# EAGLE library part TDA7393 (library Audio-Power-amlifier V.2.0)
2 x 35W Dual Bridge Car Radio Amplifier
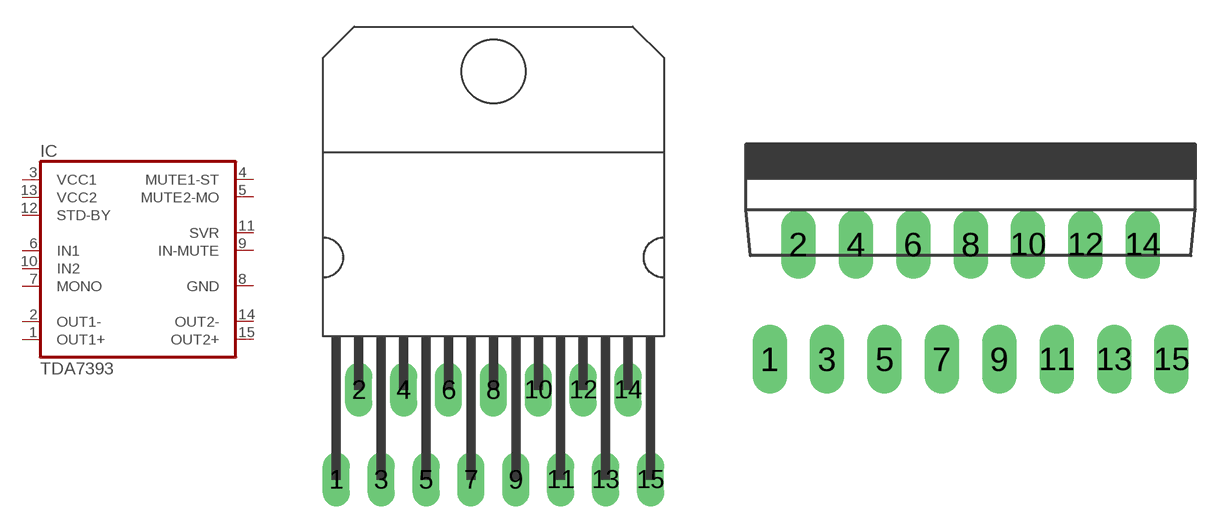
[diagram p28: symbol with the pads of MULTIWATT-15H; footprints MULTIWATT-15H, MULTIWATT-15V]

Designator prefix IC

## TDA7393H  [MULTIWATT-15H]
1  OUT1+  out
2  OUT1-  out
3  VCC1  pwr
4  MUTE1-ST  in
5  MUTE2-MO  in
6  IN1  in
7  MONO  in
8  GND  pwr
9  IN-MUTE  in
10  IN2  in
11  SVR  pas
12  STD-BY  in
13  VCC2  pwr
14  OUT2-  out
15  OUT2+  out

## TDA7393V  [MULTIWATT-15V]
Pads as for MULTIWATT-15H

## Footprint MULTIWATT-15H (pad centres in mm)
Multiwatt 15 horizontal
drill 1.016 long: 1 -8.89,-5.08; 2 -7.62,0; 3 -6.35,-5.08; 4 -5.08,0; 5 -3.81,-5.08; 6 -2.54,0; 7 -1.27,-5.08; 8 0,0; 9 1.27,-5.08; 10 2.54,0; 11 3.81,-5.08; 12 5.08,0; 13 6.35,-5.08; 14 7.62,0; 15 8.89,-5.08

## Footprint MULTIWATT-15V (pad centres in mm)
Multiwatt 15 vertical
drill 1.016 long: 1 -8.89,-5.08; 2 -7.62,0; 3 -6.35,-5.08; 4 -5.08,0; 5 -3.81,-5.08; 6 -2.54,0; 7 -1.27,-5.08; 8 0,0; 9 1.27,-5.08; 10 2.54,0; 11 3.81,-5.08; 12 5.08,0; 13 6.35,-5.08; 14 7.62,0; 15 8.89,-5.08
